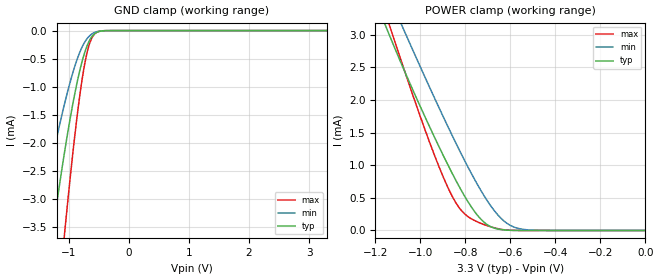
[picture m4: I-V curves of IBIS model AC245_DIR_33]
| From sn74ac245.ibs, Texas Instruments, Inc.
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[Model]   AC245_DIR_33
Model_type  Input
Vinl=0.9
Vinh=2.1
| variable   typ   min   max
C_comp   0.84pF   0.72pF   1.05pF
[Temperature Range]   40   100   -40
| Ambient temperature   25   85   -40
[Voltage range]   3.3   3   3.6
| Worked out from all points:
|   GND clamp passes 1 mA (typ) near -0.88 V on its own axis
|   POWER clamp passes 1 mA (typ) near -0.88 V on its own axis
[GND Clamp]
| AC245_DIR_33
|   Voltage   I(typ)   I(min)   I(max)
-3.3V     -25.12mA   -16.27mA   -34.01mA
-1.53V    -5.767mA   -3.652mA   -9.14mA
-1.49V    -5.414mA   -3.423mA   -8.626mA
-1.255V   -3.478mA   -2.163mA   -5.708mA
-1.08V    -2.21mA    -1.334mA   -3.692mA
-1.05V    -2.01mA    -1.204mA   -3.365mA
-920mV    -1.22mA    -696.7uA   -2.04mA
-785mV    -567uA     -303uA     -902.5uA
-680mV    -227.3uA   -120.6uA   -317.7uA
-580mV    -62.52uA   -37.32uA   -70.18uA
-380mV    -1.689uA   -1.223uA   -888.1nA
3.3V      4.213nA    12.06nA    20.26nA
[POWER Clamp]
| AC245_DIR_33
|   Voltage   I(typ)   I(min)   I(max)
-3.3V     25.79mA    24.73mA    28.42mA
-1.145V   3.061mA    3.64mA     3.232mA
-1.12V    2.852mA    3.443mA    2.968mA
-1.09V    2.605mA    3.208mA    2.655mA
-1.065V   2.405mA    3.012mA    2.398mA
-900mV    1.165mA    1.759mA    836.2uA
-840mV    755.6uA    1.327mA    415uA
-785mV    423.5uA    951.8uA    204.9uA
-695mV    72.52uA    417uA      64.94uA
-630mV    9.041uA    150.1uA    12.41uA
-575mV    1.283uA    41.58uA    638.1nA
-48.03fV  4.213nA    632.2pA    31.47nA
